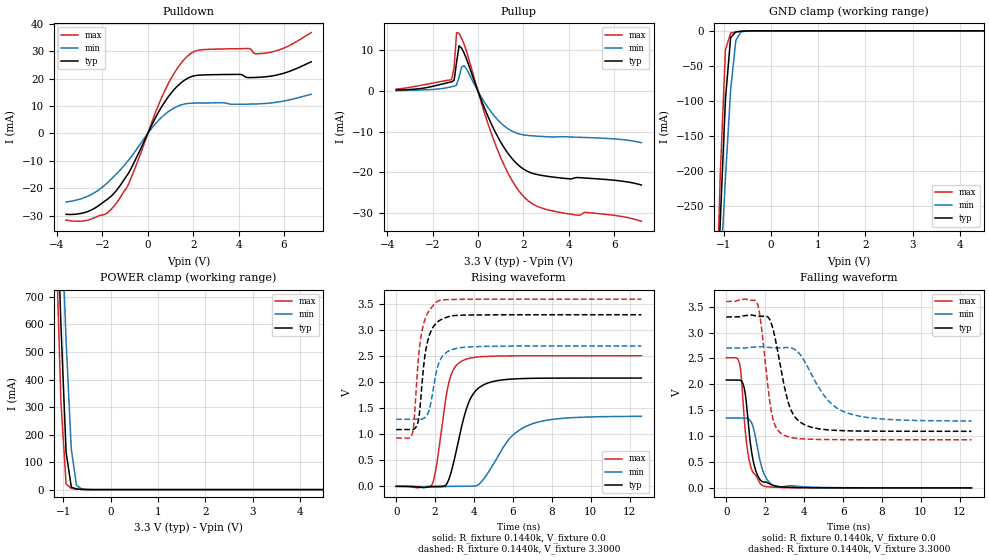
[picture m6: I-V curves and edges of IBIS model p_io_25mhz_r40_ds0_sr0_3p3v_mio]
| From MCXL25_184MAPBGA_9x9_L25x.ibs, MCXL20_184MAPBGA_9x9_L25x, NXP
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[Model] p_io_25mhz_r40_ds0_sr0_3p3v_mio
|   Model p_io_25mhz_r40_ds0_sr0_3p3v_mio
| This model was characterised for following simulation conditions:
| External (pad) voltage:
|   - Typ: 3.3V,   - Min: 2.7V,   - Max: 3.6V
| Library cells for typ/min/max conditions are connected as defined below:
|  pad - External Pad
|  ipp_do_lv - Core Input
|  ipp_obe_lv - Output Buffer Enable
|  IOGC - NC
|  REFH3V3 - REFH3V3
|  REFL3V3 - REFL3V3
|  ZI - NC
|  abut_ncal_vddio[1] - vddio
|  abut_ncal_vddio[2] - vddio
|  abut_ncal_vddio[3] - vssio
|  abut_ncal_vddio[4] - vddio
|  abut_ncal_vddio[5] - vddio
|  abut_ncal_vddio[6] - vssio
|  abut_pcal_vddio[1] - vssio
|  abut_pcal_vddio[2] - vssio
|  abut_pcal_vddio[3] - vddio
|  abut_pcal_vddio[4] - vssio
|  abut_pcal_vddio[5] - vssio
|  abut_pcal_vddio[6] - vddio
|  ipp_do_1p8v - ipp_do_1p8v
|  ipp_dse_lv - 0
|  ipp_eftd_lv - NC
|  ipp_ina_mux_vddio - NC
|  ipp_ina_mux_vddio[0] - NC
|  ipp_ina_mux_vddio[1] - NC
|  ipp_ina_r0_vddio - NC
|  ipp_ina_r0a_vddio - NC
|  ipp_ina_r0b_vddio - NC
|  ipp_ina_r0c_vddio - NC
|  ipp_ina_r0d_vddio - NC
|  ipp_ina_r0e_vddio - NC
|  ipp_ina_r0f_vddio - NC
|  ipp_ina_r300_vddio - NC
|  ipp_ina_r300a_vddio - NC
|  ipp_ina_r300b_vddio - NC
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Model_type I/O
Polarity   Non-Inverting
Enable   Active-High
Vinl =   0.9900V
Vinh =   2.3100V
Vmeas =  1.6500V
Cref =   30.0000pF
Rref =   1.0000M
Vref =   3.3000V
C_comp   1.6860pF   1.6265pF   1.7672pF
|C_comp_pullup   0.5961pF   0.6271pF   0.5748pF
|C_comp_pulldown   0.8295pF   0.8779pF   0.7919pF
[Model Spec]
| variable   typ   min   max
Vinh   2.3100V   1.8900V   2.5200V
Vinl   0.9900V   0.8100V   1.0800V
[Temperature Range]   25.0000   0.1250k   -40.0000
[Voltage Range]   3.3000V   2.7000V   3.6000V
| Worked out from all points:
|   slope of the pulldown table from 0 to 0.495 V, typ, clamps not added: 61.3 ohm
|   slope of the pullup table from 0 to 0.495 V, typ, clamps not added: 71.6 ohm
|   GND clamp passes 1 mA (typ) near -0.67 V on its own axis
|   POWER clamp passes 1 mA (typ) near -0.62 V on its own axis
|   rising waveform, R_fixture 0.1440k, V_fixture 0.0: 20-80 % time 864ps typ, 1.58ns min, 600ps max; typ from 0 V to 2.08 V
|   rising waveform, R_fixture 0.1440k, V_fixture 3.3000: 20-80 % time 436ps typ, 483ps min, 412ps max; typ from 1.09 V to 3.3 V
|   falling waveform, R_fixture 0.1440k, V_fixture 0.0: 20-80 % time 424ps typ, 497ps min, 395ps max; typ from 2.08 V to 0 V
|   falling waveform, R_fixture 0.1440k, V_fixture 3.3000: 20-80 % time 766ps typ, 1.5ns min, 500ps max; typ from 3.3 V to 1.09 V
[Pulldown]
|Voltage   I(typ)   I(min)   I(max)
-3.6V     -29.47mA   -24.96mA   -31.54mA
-2.5V     -27.93mA   -22.28mA   -31.2mA
-1.84V    -24.33mA   -18.43mA   -29.28mA
-1.4V     -20.95mA   -14.9mA    -25.56mA
-850mV    -14.52mA   -9.754mA   -18.49mA
800mV     12.14mA    7.26mA     16.44mA
1.35V     17.6mA     10.02mA    24.3mA
1.9V      20.64mA    10.99mA    29.15mA
4.43V     20.33mA    10.66mA    30.92mA
4.76V     20.39mA    10.73mA    29mA
5.31V     20.74mA    11.01mA    29.43mA
7.2V      26.08mA    14.26mA    36.73mA
[Pullup]
|Voltage   I(typ)   I(min)   I(max)
-3.6V     251.1uA    138.4uA    485.1uA
-1.16V    2.273mA    1.07mA     2.803mA
-1.05V    2.605mA    1.214mA    5.78mA
-940mV    7.098mA    1.466mA    14.39mA
-830mV    11.13mA    3.483mA    14.16mA
-720mV    10.55mA    5.906mA    12.99mA
-610mV    9.34mA     6.201mA    11.54mA
820mV     -10.68mA   -6.751mA   -13.85mA
1.48V     -16.44mA   -9.786mA   -21.76mA
2.03V     -19.26mA   -10.79mA   -26.02mA
3.35V     -21.17mA   -11.31mA   -29.54mA
7.2V      -23.1mA    -12.68mA   -32.02mA
[GND_clamp]
|Voltage   I(typ)   I(min)   I(max)
-3.6V     -5.343A    -4.159A    -6.913A
-1.18V    -470.5mA   -501mA     -462.9mA
-1.07V    -274.4mA   -353mA     -207.6mA
-960mV    -98.09mA   -211.4mA   -27.2mA
-850mV    -9.59mA    -84.32mA   -3.159mA
-740mV    -1.542mA   -13.52mA   -1.688mA
-630mV    -656uA     -1.44mA    -722.1uA
-300mV    -859.4nA   -5.611uA   -163.9nA
7.2V      0A         0A         0A
[POWER_clamp]
|Voltage   I(typ)   I(min)   I(max)
-3.6V     14.48A     12.95A     16.35A
-1.16V    1.177A     1.535A     951.2mA
-1.05V    598.4mA    1.032A     318mA
-940mV    134.2mA    537.3mA    20.05mA
-830mV    8.719mA    145.4mA    4.267mA
-720mV    2.135mA    15.38mA    2.236mA
-610mV    852.8uA    1.854mA    844.7uA
7.2V      0A         0A         0A
[Ramp]
| variable   typ   min   max
dV/dt_r  1.2495/0.8637n   0.8078/1.5783n   1.5064/0.5999n
dV/dt_f  1.3249/0.7661n   0.8453/1.5046n   1.6024/0.5003n
R_load = 0.1440k
[Rising Waveform]
R_fixture= 0.1440k
V_fixture= 0.0
V_fixture_min= 0.0
V_fixture_max= 0.0
|time   V(typ)   V(min)   V(max)
0s        4.64nV     156.5nV    15.82nV
1.84ns    -3.738mV   -13.63mV   34.02mV
2.072ns   -158.3uV   -16.65mV   401.8mV
2.691ns   121.4mV    -1.332mV   1.975V
3.395ns   1.203V     896.7uV    2.414V
3.791ns   1.669V     1.231mV    2.464V
4.353ns   1.923V     78.16mV    2.493V
5.83ns    2.06V      921.9mV    2.509V
6.892ns   2.077V     1.189V     2.51V
12.6ns    2.083V     1.346V     2.511V
[Rising Waveform]
R_fixture= 0.1440k
V_fixture= 3.3000
V_fixture_min= 2.7000
V_fixture_max= 3.6000
|time   V(typ)   V(min)   V(max)
0s        1.092V     1.289V     929.3mV
827.3ps   1.091V     1.289V     1.012V
919.8ps   1.103V     1.289V     1.256V
1.084ns   1.191V     1.289V     2.218V
1.275ns   1.739V     1.29V      2.884V
1.547ns   2.677V     1.352V     3.276V
2.109ns   3.157V     2.269V     3.555V
2.504ns   3.239V     2.554V     3.588V
3.382ns   3.292V     2.67V      3.596V
12.6ns    3.3V       2.7V       3.6V
[Falling Waveform]
R_fixture= 0.1440k
V_fixture= 0.0
V_fixture_min= 0.0
V_fixture_max= 0.0
|time   V(typ)   V(min)   V(max)
0s        2.083V     1.348V     2.511V
631.2ps   2.083V     1.348V     2.454V
744.2ps   2.074V     1.348V     2.241V
865.9ps   1.998V     1.349V     1.631V
1.016ns   1.687V     1.349V     943.5mV
1.213ns   930.9mV    1.307V     467.3mV
1.478ns   373.9mV    1.016V     261mV
1.853ns   119.3mV    358.3mV    45mV
2.739ns   21.55mV    20.45mV    7.362mV
12.6ns    217.4nV    14.99uV    44.4nV
[Falling Waveform]
R_fixture= 0.1440k
V_fixture= 3.3000
V_fixture_min= 2.7000
V_fixture_max= 3.6000
|time   V(typ)   V(min)   V(max)
0s        3.3V       2.7V       3.6V
1.581ns   3.317V     2.722V     3.573V
1.775ns   3.311V     2.725V     3.194V
2.314ns   3.174V     2.708V     1.47V
2.904ns   2.101V     2.706V     1.029V
3.271ns   1.552V     2.706V     977mV
3.743ns   1.285V     2.599V     950.5mV
5.011ns   1.128V     1.79V      933.1mV
6.099ns   1.103V     1.462V     930.5mV
12.6ns    1.092V     1.291V     929.3mV
